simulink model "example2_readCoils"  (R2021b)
settings: Solver=FixedStepDiscrete  StartTime=0.0  StopTime=10.0  FixedStep=0.8  RelTol=1e-3
libraries: ModbusServerLib x3

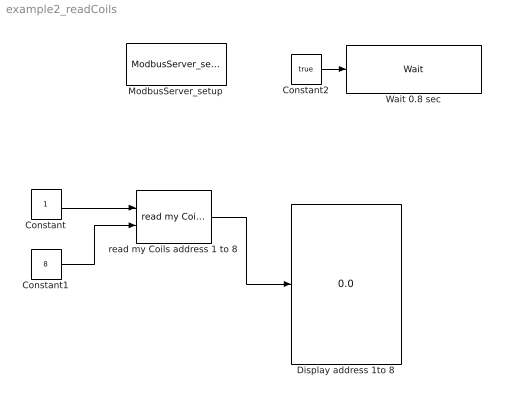
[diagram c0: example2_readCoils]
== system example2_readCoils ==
  Constant : Constant
  Constant1 : Constant  Value=8
  Constant2 : Constant  Value=true
  Display address 1to 8 : Display
  ModbusServer_setup : ModbusServerLib/ModbusServer_setup  g1_cmbPortName="\"COM5\""  g2_cmbModbusType="\"Modbus TCP\""  g3_chkIgnoreServerID=off  g4_ObjectID=0  g5_ServerID=1  g30_TCPPort=502  g6_chkSupportDINCoil1to4=on  g7_HoldingRegsSeg1to4=[ 1,30 ; 35, 56]  g8_InputRegsSeg1to4=[1 44; 78 89]  g9_CoilSeg1to4=[1 44; 78 89]  g10_DiscreteSeg1to4=[1 44; 78 89]  g11_chkUseHoldingRegstoReplace1to4=off  g12_chkEnableWD1to4=off  g13_chkUseReadonlyRegs4WD1to4=off  g14_WDAddr1to4=1  g15_cmbWDType1to4=0  g16_WDPeriod1to4=20  g17_WDPreset1to4=20  g18_chkSupportDINCoil5=on  g19_HoldingRegsSeg5=[ 1,30 ; 35, 56]  g20_InputRegsSeg5=[1 44; 78 89]  g21_CoilSeg5=[1 44; 78 89]  g22_DiscreteSeg5=[1 44; 78 89]  g23_chkUseHoldingRegstoReplace5=off  g24_chkEnableWD5=off  g25_chkUseReadonlyRegs4WD5=off  g26_WDAddr5=1  g27_cmbWDType5=0  g28_WDPeriod5=20  g29_WDPreset5=20
  Wait 0.8 sec : ModbusServerLib/Wait  Waitms=800
  read my Coils address 1 to 8 : ModbusServerLib/read my Coils  g_ObjID=0  g_DeviceNum=1
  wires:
  Constant/1 -> read my Coils address 1 to 8/1
  Constant1/1 -> read my Coils address 1 to 8/2
  Constant2/1 -> Wait 0.8 sec/1
  read my Coils address 1 to 8/1 -> Display address 1to 8/1
